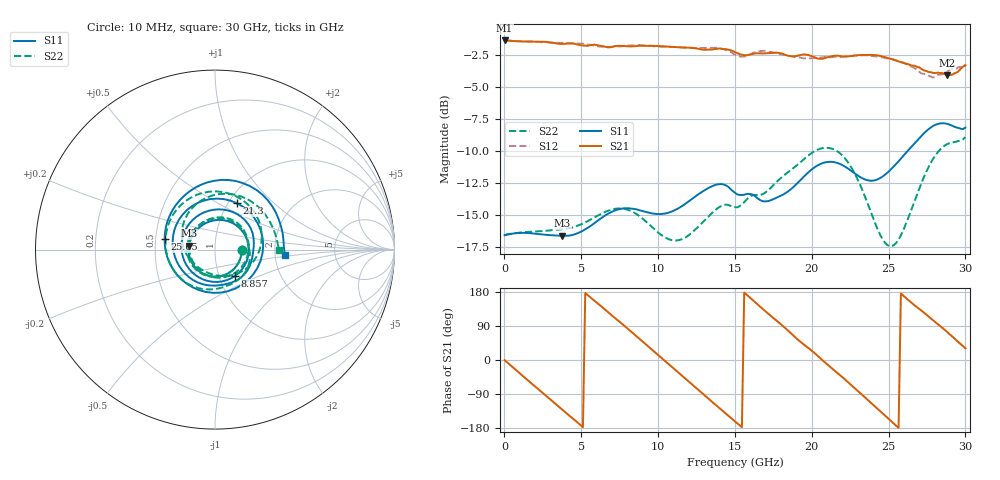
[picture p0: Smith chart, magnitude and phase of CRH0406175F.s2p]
#HZ S MA R 50
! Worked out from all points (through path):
!   201 points, 10 MHz to 30 GHz, reference 50 ohm
!   highest |S21| = -1.39 dB at 10 MHz (marker M1); lowest = -4.1 dB at 28.8 GHz (marker M2)
!   group delay of S21, straight-line fit = 97.2 ps
!   lowest |S11| = -16.7 dB at 3.759 GHz (marker M3), VSWR 1.34, Z = 37.3 + j1.62 ohm
!   |S11| at or under -10 dB: start of sweep to 26.26 GHz
!   |S22| runs from -17.5 to -8.9 dB; largest |S21 - S12| = 0.039
!   S11 on the Smith chart (normalised r, x): 10 MHz: 1.35, -0.00; 8.857 GHz: 1.19, -0.36; 21.3 GHz: 1.10, +0.62; 25.65 GHz: 0.56, +0.07; 30 GHz: 2.26, -0.15
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1e7  0.1478 -0.5  0.8522 -0.4  0.852 -0.4  0.1477 -0.4
1.95935e9  0.1499 -100.0  0.8429 -68.6  0.8428 -68.4  0.1527 -98.2
3.75875e9  0.147 -188.3  0.8259 -130.8  0.8336 -130.8  0.1561 -185.8
5.1083e9  0.1539 -243.6  0.8151 -177.3  0.8284 -176.9  0.1642 -241.4
7.2076e9  0.1848 -330.1  0.8105 -249.8  0.8045 -250.1  0.1874 -324.6
8.85705e9  0.1846 -412.6  0.8126 -306.5  0.8166 -306.3  0.1741 -401.2
1.005665e10  0.1787 -479.0  0.8096 -348.7  0.8067 -348.9  0.1506 -464.2
1.125625e10  0.1873 -543.2  0.8018 -390.9  0.8021 -390.9  0.141 -528.0
1.26058e10  0.2133 -607.2  0.7907 -437.9  0.7954 -438.7  0.1593 -593.1
1.38054e10  0.233 -661.6  0.7895 -480.5  0.7979 -480.4  0.1871 -649.2
1.5005e10  0.2164 -715.6  0.7666 -522.0  0.7502 -522.0  0.1902 -706.7
1.635455e10  0.2089 -775.8  0.7594 -569.0  0.7684 -570.0  0.2122 -772.4
1.77041e10  0.207 -838.5  0.7634 -616.0  0.7602 -615.8  0.2383 -840.7
1.875375e10  0.2266 -889.3  0.7391 -653.6  0.7387 -653.7  0.2689 -892.7
2.01033e10  0.27 -954.4  0.7359 -698.9  0.7277 -699.9  0.3126 -952.1
2.13029e10  0.2859 -1015.6  0.7389 -741.7  0.7336 -740.9  0.3222 -1005.0
2.325225e10  0.2474 -1132.8  0.7476 -810.8  0.7452 -810.6  0.2248 -1096.6
2.505165e10  0.2635 -1243.5  0.7246 -877.2  0.7242 -878.3  0.134 -1193.9
2.565145e10  0.2873 -1272.1  0.7053 -899.2  0.7072 -899.5  0.1421 -1227.8
2.715095e10  0.3618 -1332.0  0.6589 -950.0  0.6327 -947.8  0.2372 -1304.7
2.88004e10  0.4028 -1396.9  0.6232 -1005.4  0.6428 -1007.0  0.335 -1384.5
3e10  0.3892 -1444.0  0.6825 -1049.1  0.677 -1050.6  0.3572 -1440.5
